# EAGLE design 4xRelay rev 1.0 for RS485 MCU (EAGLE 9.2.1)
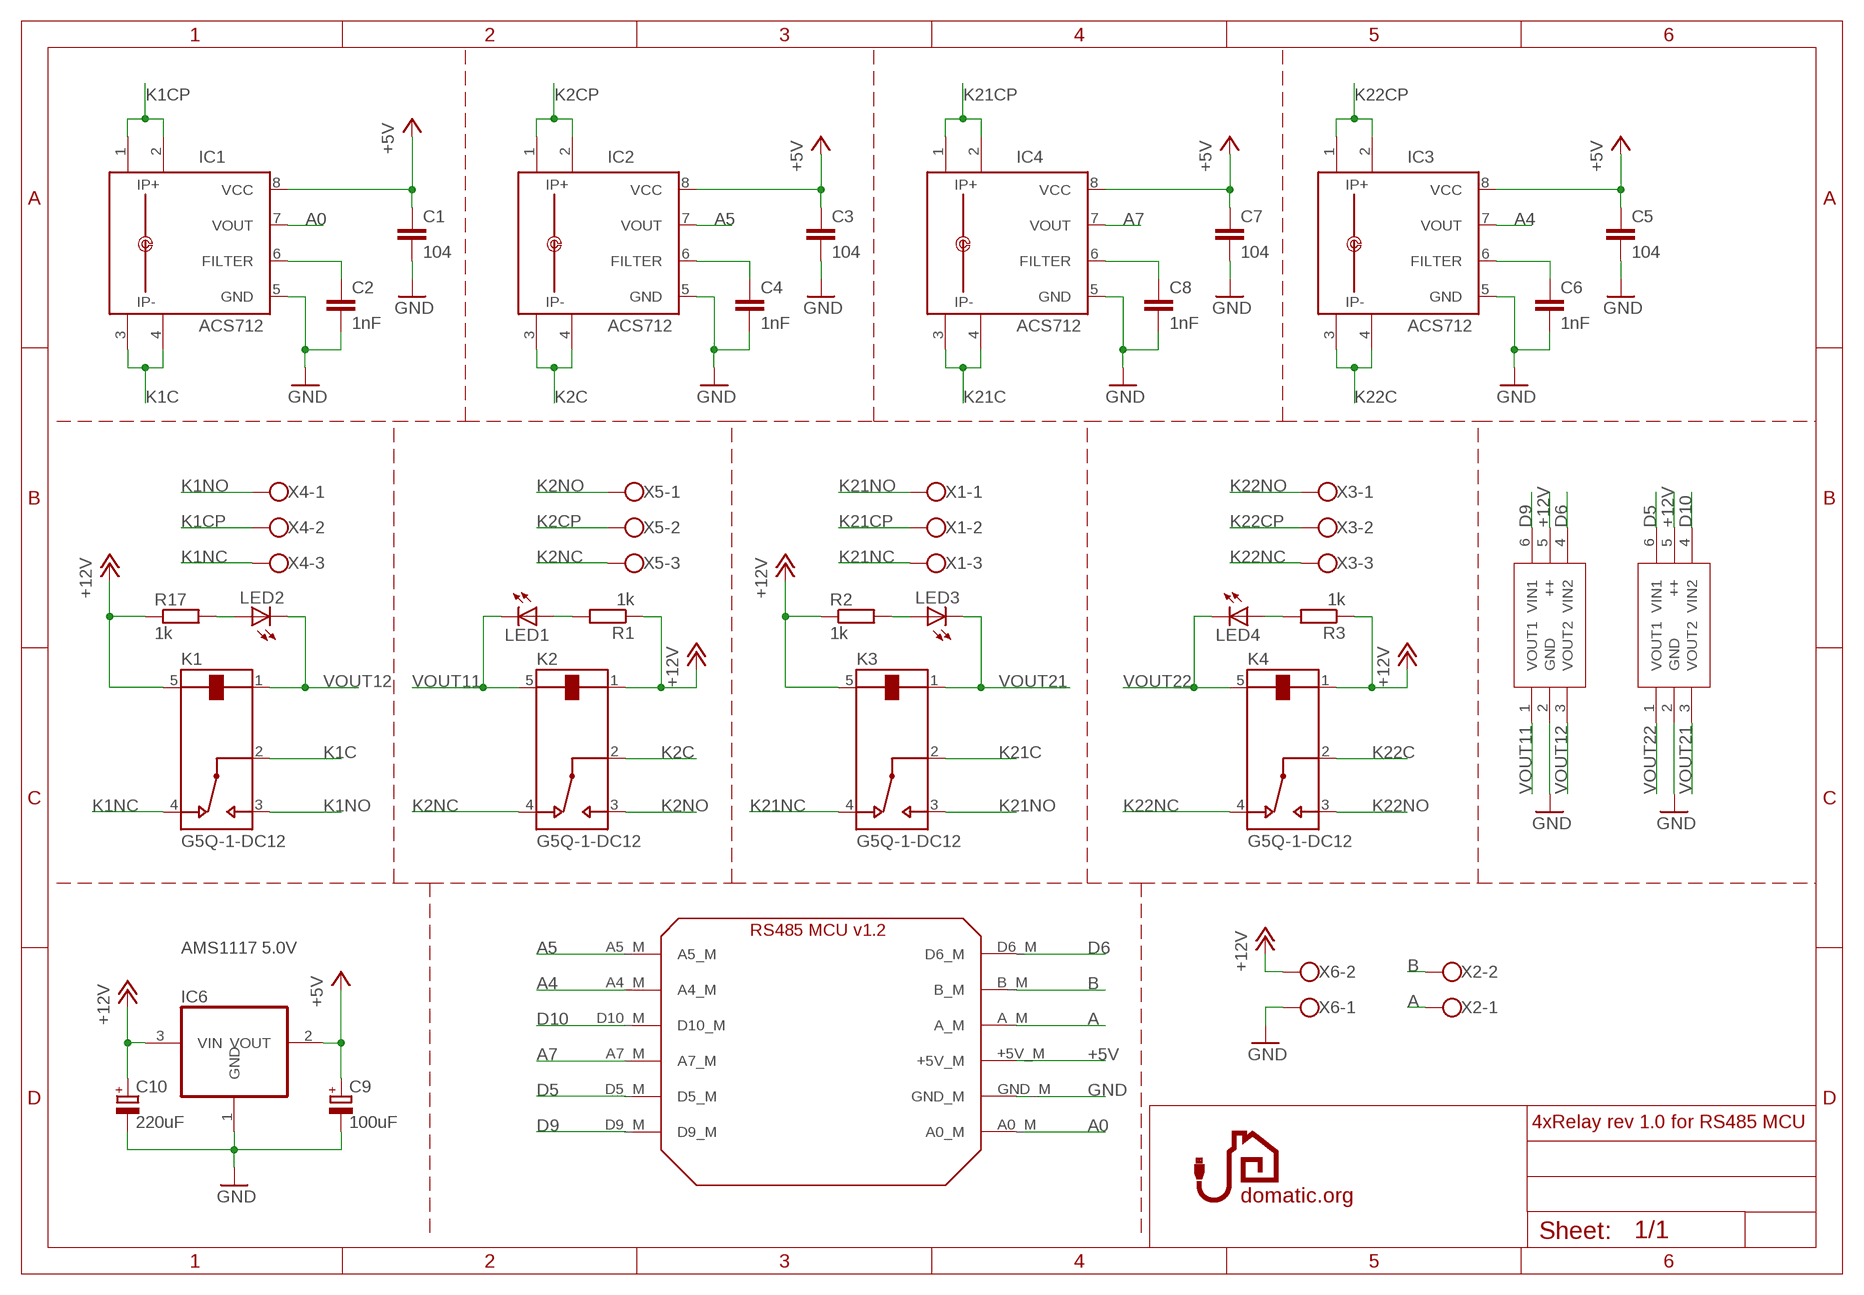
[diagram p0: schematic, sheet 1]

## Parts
C1  104  C-EUC0603  [C0603]
C2  1nF  C-EUC0603  [C0603]
C3  104  C-EUC0603  [C0603]
C4  1nF  C-EUC0603  [C0603]
C5  104  C-EUC0603  [C0603]
C6  1nF  C-EUC0603  [C0603]
C7  104  C-EUC0603  [C0603]
C8  1nF  C-EUC0603  [C0603]
C9  100uF  CPOL-EUE2.5-6  [E2,5-6]
C10  220uF  CPOL-EUE2.5-6  [E2,5-6]
IC1  ACS712  ACS712-LC  [SOIC8]
IC2  ACS712  ACS712-LC  [SOIC8]
IC3  ACS712  ACS712-LC  [SOIC8]
IC4  ACS712  ACS712-LC  [SOIC8]
IC6  AMS1117 5.0V  REG1117  [SOT223]
K1  G5Q-1-DC12  [RELAY_G5Q-1-DC12]
K2  G5Q-1-DC12  [RELAY_G5Q-1-DC12]
K3  G5Q-1-DC12  [RELAY_G5Q-1-DC12]
K4  G5Q-1-DC12  [RELAY_G5Q-1-DC12]
LED1  LEDSML0805  [SML0805]
LED2  LEDSML0805  [SML0805]
LED3  LEDSML0805  [SML0805]
LED4  LEDSML0805  [SML0805]
R1  1k  R-EU_R0603  [R0603]
R2  1k  R-EU_R0603  [R0603]
R3  1k  R-EU_R0603  [R0603]
R17  1k  R-EU_R0603  [R0603]
U$1  DRDNB21D  [DRDNB21D-7]
U$2  RS485_MCU_1.2  [RS485_MCU_V1_2_DO_SHIELD]
U$3  DRDNB21D  [DRDNB21D-7]
X1  W237-103  [W237-103]
X2  W237-102  [W237-102]
X3  W237-103  [W237-103]
X4  W237-103  [W237-103]
X5  W237-103  [W237-103]
X6  W237-102  [W237-102]

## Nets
+5V [zasilanie]: C1.1 C3.1 C5.1 C7.1 C9.+ IC1.8(VCC) IC2.8(VCC) IC3.8(VCC) IC4.8(VCC) IC6.2(VOUT) U$2.+5V_M
+12V [zasilanie]: C10.+ IC6.3(VIN) K1.5 K2.1 K3.5 K4.1 R1.1 R2.1 R3.1 R17.1 U$1.5(++) U$3.5(++) X6.2
A: U$2.A_M X2.1
A0: IC1.7(VOUT) U$2.A0_M
A4: IC3.7(VOUT) U$2.A4_M
A5: IC2.7(VOUT) U$2.A5_M
A7: IC4.7(VOUT) U$2.A7_M
B: U$2.B_M X2.2
D5: U$2.D5_M U$3.6(VIN1)
D6: U$1.4(VIN2) U$2.D6_M
D9: U$1.6(VIN1) U$2.D9_M
D10: U$2.D10_M U$3.4(VIN2)
GND [zasilanie]: C1.2 C2.2 C3.2 C4.2 C5.2 C6.2 C7.2 C8.2 C9.- C10.- IC1.5(GND) IC2.5(GND) IC3.5(GND) IC4.5(GND) IC6.1(GND) U$1.2(GND) U$2.GND_M U$3.2(GND) X6.1
K1C [230v]: IC1.3(IP-) IC1.4(IP-1) K1.2
K1CP [230v]: IC1.1(IP+) IC1.2(IP+1) X4.2
K1NC [230v]: K1.4 X4.3
K1NO [230v]: K1.3 X4.1
K2C [230v]: IC2.3(IP-) IC2.4(IP-1) K2.2
K2CP [230v]: IC2.1(IP+) IC2.2(IP+1) X5.2
K2NC [230v]: K2.4 X5.3
K2NO [230v]: K2.3 X5.1
K21C [230v]: IC4.3(IP-) IC4.4(IP-1) K3.2
K21CP [230v]: IC4.1(IP+) IC4.2(IP+1) X1.2
K21NC [230v]: K3.4 X1.3
K21NO [230v]: K3.3 X1.1
K22C [230v]: IC3.3(IP-) IC3.4(IP-1) K4.2
K22CP [230v]: IC3.1(IP+) IC3.2(IP+1) X3.2
K22NC [230v]: K4.4 X3.3
K22NO [230v]: K4.3 X3.1
N$1: LED2.A R17.2
N$2: LED1.A R1.2
N$3: LED3.A R2.2
N$4: LED4.A R3.2
N$5: C2.1 IC1.6(FILTER)
N$6: C4.1 IC2.6(FILTER)
N$7: C6.1 IC3.6(FILTER)
N$8: C8.1 IC4.6(FILTER)
VOUT11: K2.5 LED1.C U$1.1(VOUT1)
VOUT12: K1.1 LED2.C U$1.3(VOUT2)
VOUT21: K3.1 LED3.C U$3.3(VOUT2)
VOUT22: K4.5 LED4.C U$3.1(VOUT1)

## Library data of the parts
C1-C8 = resistor:C-EU: CAPACITOR, European symbol
C9 C10 = resistor:CPOL-EU: POLARIZED CAPACITOR, European symbol
IC1-IC4 = allegro-2:ACS712-LC
IC6 = burr-brown:REG1117: 800mA and 1A Low Dropout (LDO) Positive Regulator 1.8V, 2.5V, 2.85V, 3.3V, 5V, and Adj; MPN: REG1117; OC_FARNELL: 1097566; OC_NEWARK: 14P6981
K1-K4 = G5Q-1-DC12:G5Q-1-DC12: Power Relay 12VDC 5(NO)A/3(NC)DCA/10(NO)A/3(NC)ACA SPDT (( 20.3mm 10.3mm 16.2mm)) Through Hole; AVAILABILITY: Unavailable; DESCRIPTION: Power Relay 12VDC 5_NO_A/3_NC_DCA/10_NO_A/3_NC_ACA SPDT __ 20.3mm 10.3mm 16.2mm__ Through Hole; MF: Omron; MP: G5Q-1-DC12; PACKAGE: None; PRICE: None
LED1-LED4 = led:LED: LED
R1-R3 R17 = resistor:R-EU_: RESISTOR, European symbol
U$1 U$3 = DRDNB21D:DRDNB21D
U$2 = rs:RS485_MCU_1.2
X1 X3-X5 = con-wago-500:W237-103: WAGO SCREW CLAMP; MPN: 237-103; OC_FARNELL: unknown; OC_NEWARK: 18M7116
X2 X6 = con-wago-500:W237-102: WAGO SCREW CLAMP; MPN: 237-102; OC_FARNELL: unknown; OC_NEWARK: 70K9898

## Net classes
0 default: width 0.4 mm, drill 0.8 mm, clearance 0.25 mm
1 zasilanie: width 0.4 mm, drill 0.8 mm, clearance 0.25 mm
2 230v: width 0.5 mm, drill 1 mm, clearance 2 mm

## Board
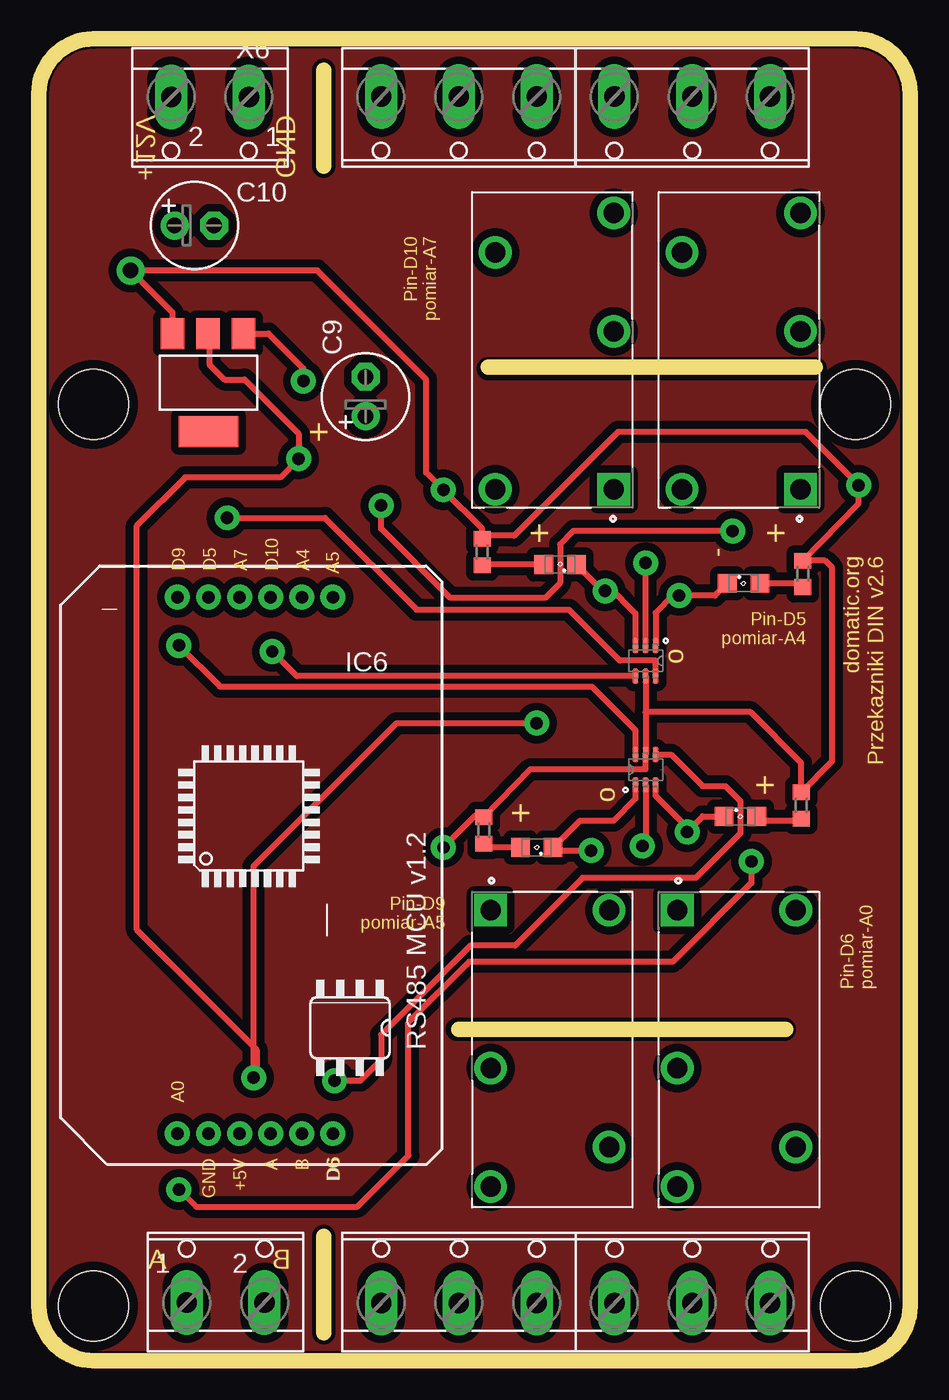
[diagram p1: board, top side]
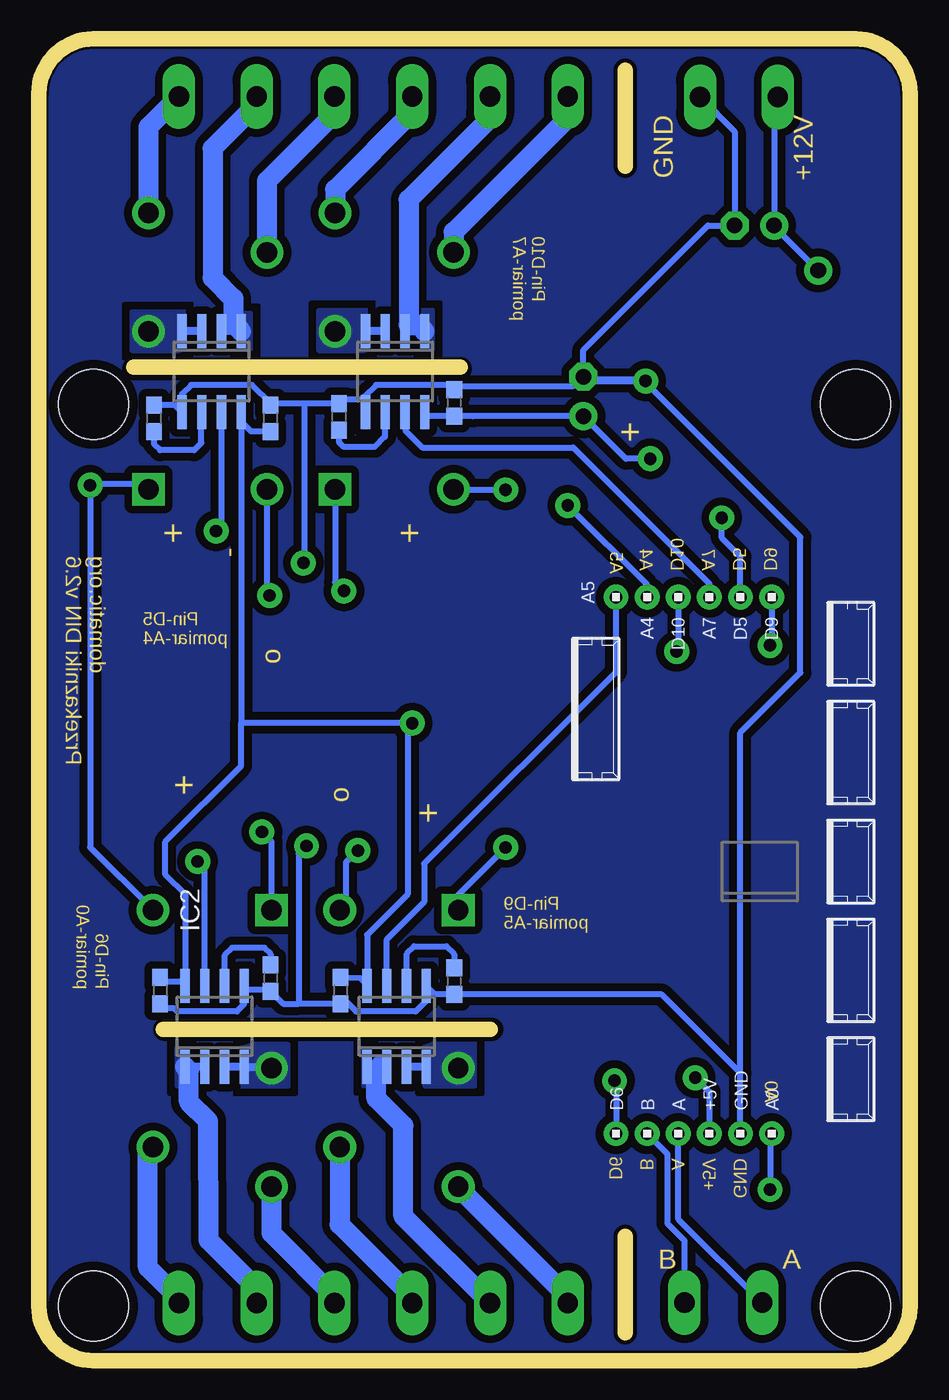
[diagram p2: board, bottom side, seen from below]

Size 56 x 85 mm. Coordinates in mm from the lower left corner, seen from the top.
Outline: 26.9,21.3 47.9,21.3
Outline: 28.9,63.8 49.9,63.8
Outline: 18.3,1.8 18.3,8
Outline: 18.3,76.8 18.3,83
Outline: 0,81.5 0,3.5 arc90 3.5,0 52.5,0 arc90 56,3.5 56,81.5 arc90 52.5,85 3.5,85 arc90 0,81.5
Copper layers (1*16): Top 0.035mm / dielectric 1.5mm / Bottom 0.035mm
Design rules "default *": minimum track width 0.3mm, minimum drill 0.8mm, track to track 0.2mm, track to pad 0.2mm, pad to pad 0.2mm, via to via 0.2mm, smd to smd 0.2mm, copper to edge 0.6mm, drill to drill 0.3mm, minimum pad ring 0.4mm, minimum via ring 0.4mm, stop-mask expansion 4mil, vias tented up to drill 0mil, thermal gap 0.4mm
Holes 4.5 mm at 52.5,61.5 3.5,61.5 52.5,3.5 3.5,3.5
Milling: 12 lines

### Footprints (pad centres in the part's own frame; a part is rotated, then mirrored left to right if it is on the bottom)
C0603 = smd 1.1 x 1: 1 -0.85,0; 2 0.85,0
E2,5-6 = drill 1 pad 1.6: + -1.27,0 | drill 1 pad 1.6 octagon: - 1.27,0
SOIC8 = smd 0.6 x 2.2: 1 -1.905,-2.6; 2 -0.635,-2.6; 3 0.635,-2.6; 4 1.905,-2.6; 5 1.905,2.6; 6 0.635,2.6; 7 -0.635,2.6; 8 -1.905,2.6
SOT223 = smd 1.499 x 2.007: 1 -2.261,-3.15; 2 0.025,-3.15; 3 2.311,-3.15 | smd 3.81 x 2.007: 4 0,3.15
RELAY_G5Q-1-DC12 = drill 1.3 square: 1 -8.97,-3.96 | drill 1.3: 2 1.19,-3.96; 3 8.81,-3.96; 4 6.27,3.66; 5 -8.97,3.66
SML0805 = smd 1.2 x 1.2: A 1.05,0; C -1.05,0
R0603 = smd 1 x 1.1: 1 -0.85,0; 2 0.85,0
DRDNB21D-7 = smd 0.97 x 0.39: 1 -0.98,0.65; 2 -0.98,0; 3 -0.98,-0.65; 4 0.98,-0.65; 5 0.98,0; 6 0.98,0.65
RS485_MCU_V1_2_DO_SHIELD = drill 0.8 pad 1.422: +5V_M 36.5,12; A0_M 36.5,8; A4_M 2,16; A5_M 2,18; A7_M 2,12; A_M 36.5,14; B_M 36.5,16; D5_M 2,10; D6_M 36.5,18; D9_M 2,8; D10_M 2,14; GND_M 36.5,10
W237-103 = drill 1.3 long: 1 -5,-1.29; 2 0,-1.29; 3 5,-1.29
W237-102 = drill 1.3 long: 1 -2.5,-1.27; 2 2.5,-1.27

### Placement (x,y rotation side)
C1  48.2,23.8 270 bottom
C2  41.1,24.6 270 bottom
C3  36.6,23.8 270 bottom
C4  29.3,24.4 270 bottom
C5  41.1,60.6 90 bottom
C6  48.6,60.6 90 bottom
C7  29.3,61.6 90 bottom
C8  36.7,60.7 90 bottom
C9  21,62 90 top
C10  10,73 0 top
IC1  44.7,21.5 0 bottom
IC2  33,21.5 0 bottom
IC3  44.9,63.6 180 bottom
IC4  33.1,63.6 180 bottom
IC6  10.9,62.9 180 top
K1  45,20 270 top
K2  33,20 270 top
K3  33,65 90 top
K4  45,65 90 top
LED1  32,33 180 top
LED2  45.1,35 0 top
LED3  33.5,51.2 180 top
LED4  45.3,50 0 top
R1  28.6,34.1 270 top
R2  28.5,52 270 top
R3  49.1,50.6 270 top
R17  49,35.7 270 top
U$1  39,38 90 top
U$2  0.9,51.1 270 top
U$3  39,45 270 top
X1  27,80 180 top
X2  12,5 0 top
X3  42,80 180 top
X4  42,5 0 top
X5  27,5 0 top
X6  11,80 180 top

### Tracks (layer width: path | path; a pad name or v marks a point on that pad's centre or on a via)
+5V  (via drill 0.8)
  Top 0.4: v32,41 23,41 13.8,31.8 v13.8,18.2 14,18.39 14,20 6.3,27.7 6.3,53.7 9.4,56.8 15.5,56.8 v16.7,58 16.7,59.62 13.23,63.1 11.93,63.1 10.96,64.06 10.96,65.96 IC6.2
  Bottom 0.4: IC4.8 31.2,60.75 C7.1 29.28,60.73 28.08,60.73 28.06,60.75 21.02,60.75 C9.+ 18.27,58 v16.7,58 | C5.1 42.35,59.75 42.99,60.4 IC3.8 42.99,41 | 34.92,24.2 35.33,24.61 C3.1 36.7,24.7 36.68,24.72 36.66,24.7 C3.1 | 34.92,24.2 34.86,24.14 | v13.8,18.2 12.9,17.29 U$2.+5V_M | C1.1 47.95,24.4 46.91,24.4 IC1.8 46.6,29.98 47.86,31.24 47.86,33.38 42.99,38.24 42.99,41 | 42.99,41 v32,41 32.3,40.7 32.3,29.99 34.91,27.39 IC2.8 34.91,24.21 34.92,24.2
+12V  (via drill 0.8, 1)
  Top 0.4: 39,41.7 45.75,41.7 49,38.45 R17.1 51,38.55 51,51 50.55,51.45 R3.1 52.7,55.15 v52.7,56.3 49.27,59.73 37.24,59.73 30.56,53.05 28.6,53.05 R2.1 28.5,53.5 v26,56 24.9,57.1 24.9,63.1 17.9,70.1 v5.9,70.1 8.59,67.41 IC6.3 | U$3.5 39,41.7 | 39,41.7 U$1.5 39,38.05 31.59,38.05 R1.1 28.05,35.05 v26,33
  Bottom 0.4: v26,56 29.31,56 K3.5 | K4.1 49.33,56.4 52.6,56.4 v52.7,56.3 52.7,33.01 K1.5 | X6.2 8.73,81.04 C10.+ 8.73,72.93 v5.9,70.1 | v26,33 29.04,29.96 K2.1
A
  Bottom 0.4: 14.89,14.46 14.89,9.1 9.53,3.74 | 14.89,14.46 U$2.A_M | 9.53,3.74 X2.1 | U$2.A_M 14.93,14.62 14.89,14.46 | 9.53,3.74 9.56,3.74 X2.1
A0  (via drill 0.8)
  Top 0.4: v9,11 10.1,9.9 20.47,9.9 23.75,13.18 23.75,21.75 27.65,25.65 40.74,25.65 45.8,30.71 v45.8,32.1
  Bottom 0.4: U$2.A0_M 9,14.5 v9,11 | IC1.7 45.34,31.64 v45.8,32.1
A4  (via drill 0.8)
  Top 0.4: v44.6,53.35 34.36,53.35 33.5,52.49 33.5,50.01 32.54,49.05 26.45,49.05 22,53.5 v22,55
  Bottom 0.4: IC3.7 44.27,53.69 44.49,53.46 | 44.49,53.46 v44.6,53.35 | v44.6,53.35 | v22,55 16.9,49.9 U$2.A4_M | 44.49,53.46 44.5,53.46 v44.6,53.35
A5
  Bottom 0.4: IC2.7 33.63,27.1 31.23,29.5 31.23,31.96 18.9,44.3 U$2.A5_M
A7
  Bottom 0.4: IC4.7 32.45,60.98 32.45,59.81 31.36,58.73 21.66,58.73 12.9,49.97 U$2.A7_M
B
  Bottom 0.4: X2.2 14.5,7.72 15.59,8.81 15.59,13.29 U$2.B_M
D5  (via drill 0.8)
  Top 0.4: v12.1,54.2 18.38,54.2 24.28,48.3 34.07,48.3 37.35,45.02 39.65,45.02 U$3.6
  Bottom 0.4: U$2.D5_M 10.9,51.7 12.1,52.9 v12.1,54.2
D6  (via drill 0.8)
  Top 0.4: v19,18 20.67,18 22,19.33 22,20.95 27.75,26.7 30.61,26.7 34.96,31.05 42.24,31.05 45.1,33.91 45.1,35.99 44.13,36.95 42.67,36.95 40.65,38.98 U$1.4
  Bottom 0.4: v19,18 18.9,17.9 U$2.D6_M
D9  (via drill 0.8)
  Top 0.4: v9,46 11.65,43.35 35.55,43.35 38.35,40.55 U$1.6
  Bottom 0.4: U$2.D9_M 8.9,46.1 v9,46
D10  (via drill 0.8)
  Top 0.4: U$3.4 16.58,44.02 v15,45.6
  Bottom 0.4: U$2.D10_M 14.9,45.7 v15,45.6
GND  (via drill 0.8)
  Top 0.4: U$1.2 39,33.3 v38.8,33.1 | U$3.2 v39,51.3 | IC6.1 14.75,66.05 17,63.8 v17,63
  Bottom 0.4: 35.07,62 34.32,62.75 29.6,62.75 C7.2 29.1,62.65 21.7,62.65 21.04,63.31 C9.- | 35.07,62 35.27,61.8 36.45,61.8 C8.2 38.94,61.55 | 35.07,62 34.96,62 34.96,61.1 | 31.1,24.1 31.12,24.58 31.12,24.21 | 31.12,24.21 31.12,23.11 31.78,22.45 35.6,22.45 36.35,23.2 C3.2 39.3,22.95 | 39.3,22.95 40.3,22.95 C2.2 41.2,23.85 42.55,23.85 IC1.5 42.71,23.89 42.81,23.89 | v38.8,33.1 39.3,32.6 39.3,22.95 | 34.96,61.1 34.96,61.05 IC4.5 | 42.81,23.89 42.81,24.28 IC1.5 | 42.81,23.89 42.81,22.91 43.28,22.45 47.09,22.45 47.29,22.65 47.9,22.65 C1.2 | C6.2 47.26,61.45 IC3.5 46.78,61.02 46.78,62.19 46.22,62.75 42.31,62.75 41.1,61.54 C5.2 41,61.55 38.94,61.55 | 38.94,61.55 38.94,51.3 v39,51.3 | X6.1 11.27,79.04 C10.- 13,73 21,65 C9.- | v17,63 17.1,63.1 20.83,63.1 C9.- | C9.- 20.68,62.95 17.04,62.95 7.05,52.96 7.05,44.24 10.9,40.39 U$2.GND_M 10.9,18.5 15.95,23.55 C4.2 30.55,23.55 IC2.5 31.17,24.21 31.12,24.21 | IC4.5 35.08,61.1 34.96,61.1
K1C
  Bottom 0.5: K1.2 41.09,18.85 42.55,18.85 IC1.4 IC1.3
  pour Bottom (rank 2, no thermals): 40,17.7 40,20.3 44.2,20.3 44.2,17.7
K1CP
  Bottom 0.5: IC1.2 IC1.1
  Bottom 1.27: X4.2 42,4.66 45.08,7.74 45.12,15.42 46.35,16.65 46.35,18.65 IC1.1
  pour Bottom (no thermals): 45.1,20.4 47.1,20.4 47.1,17.7 45.1,17.7
K1NC
  Bottom 1.27: X4.3 47,4 49,6 49,13.39 K1.4
K1NO
  Bottom 1.27: K1.3 41.04,8.19 37,4.15 X4.1
K2C
  Bottom 0.5: IC2.4 IC2.3
  pour Bottom (no thermals): 32.5,17.7 28,17.7 28,20.5 32.5,20.5
K2CP
  Bottom 0.5: 34,19 33.61,18.85 IC2.2 IC2.1 34.75,18.85 34.3,18.7
  Bottom 1.27: X5.2 32.58,9.29 32.58,15.12 34.3,16.85 34.3,18.7 34,19
  pour Bottom (rank 2, no thermals): 33.4,20.7 33.4,17.7 35.1,17.7 35.1,20.7
K2NC
  Bottom 1.27: K2.4 36.66,8.76 32,4.1 X5.3
K2NO
  Bottom 1.27: X5.1 22,4.1 29.04,11.14 K2.3
K21C
  Bottom 0.5: IC4.3 IC4.4
  pour Bottom (no thermals): 38,65 33.6,65 33.6,67.5 38,67.5
K21CP
  Bottom 0.5: 32.23,66.6 32.48,66.3 IC4.2 IC4.1
  Bottom 1.27: X1.2 27,79.9 32.23,74.67 32.23,66.6 31.59,66.6 IC4.1
  pour Bottom (rank 2, no thermals): 33,65 30.7,65 30.7,67.5 33,67.5
K21NC
  Bottom 1.27: X1.3 22,79.91 29.34,72.57 K3.4
K21NO
  Bottom 1.27: X1.1 32,80.27 36.96,75.31 K3.3
K22C
  Bottom 0.5: IC3.3 IC3.4
  pour Bottom (no thermals): 50,65 45.4,65 45.4,67.4 50,67.4
K22CP
  Bottom 0.5: 43.49,66.7 44.01,66.46 44.17,66.3 IC3.2 IC3.1
  Bottom 1.27: IC3.1 43.49,66.7 43.49,68.3 44.83,69.63 44.83,77.97 42,80.79 X3.2
  pour Bottom (rank 2, no thermals): 44.5,65 42.4,65 42.4,67.3 44.5,67.3
K22NC
  Bottom 1.27: X3.3 37,80.19 41.34,75.85 K4.4
K22NO
  Bottom 1.27: X3.1 48.96,79.33 K4.3
N$1
  Top 0.4: LED2.A 46.45,34.7 48.95,34.7 R17.2
N$2
  Top 0.4: LED1.A 28.75,33 R1.2
N$3
  Top 0.4: LED3.A 28.65,51.2 R2.2
N$4
  Top 0.4: 46.7,49.65 LED4.A 48.85,50 R3.2
N$5
  Bottom 0.4: IC1.6 44.05,24.12 44.05,26.09 43.58,26.55 41.5,26.55 41.1,26.15 C2.1
N$6
  Bottom 0.4: IC2.6 32.34,24.12 32.34,26.19 31.88,26.65 29.8,26.65 29.3,26.15 C4.1
N$7
  Bottom 0.4: IC3.6 45.55,60.98 45.55,59.01 46.02,58.55 48.2,58.55 48.6,58.95 C6.1
N$8
  Bottom 0.4: IC4.6 33.76,60.98 33.76,59.41 34.42,58.75 36.4,58.75 36.7,59.05 C8.1
N$9
  pour Bottom (isolate 0.5, rank 6): 0,81.5 0,3.5 arc90 3.5,0 52.5,0 arc90 56,3.5 56,81.5 arc90 52.5,85 3.5,85 arc90
N$10
  pour Top (isolate 0.5, rank 6): 0,81.5 0,3.5 arc90 3.5,0 52.5,0 arc90 56,3.5 56,81.5 arc90 52.5,85 3.5,85 arc90
VOUT11  (via drill 0.8)
  Top 0.4: U$1.1 38.35,36.12 36.95,34.72 34.77,34.72 LED1.C 33.25,32.8 v35.5,32.8 35.4,32.8
  Bottom 0.4: v35.5,32.8 36.26,32.04 36.26,29.37 K2.5
VOUT12  (via drill 0.8)
  Top 0.4: U$1.3 39.65,36.32 41.67,34.3 v41.67,34 42.67,35 LED2.C
  Bottom 0.4: K1.1 41.04,33.37 v41.67,34
VOUT21  (via drill 0.8)
  Top 0.4: LED3.C 36.25,49.5 v36.4,49.5 36.65,49.75 38.35,48.05 U$3.3
  Bottom 0.4: K3.1 36.96,50.06 v36.4,49.5
VOUT22  (via drill 0.8)
  Top 0.4: LED4.C 43.45,49.2 v41.16,49.2 40.76,49.2 39.65,48.09 U$3.1
  Bottom 0.4: K4.5 41.34,49.38 v41.16,49.2

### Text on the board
tNames: D6
Milling: +12V | GND | Pin-D10 / pomiar-A7 | + | + | + | - | domatic.org / Przekazniki DIN v2.6 | D9 | D5 | A7 | D10 | A4 | A5 | o | Pin-D5 / pomiar-A4 | + | o | + | Pin-D9 / pomiar-A5 | Pin-D6 / pomiar-A0 | A0 | GND | +5V | A | B | D6 | A | B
